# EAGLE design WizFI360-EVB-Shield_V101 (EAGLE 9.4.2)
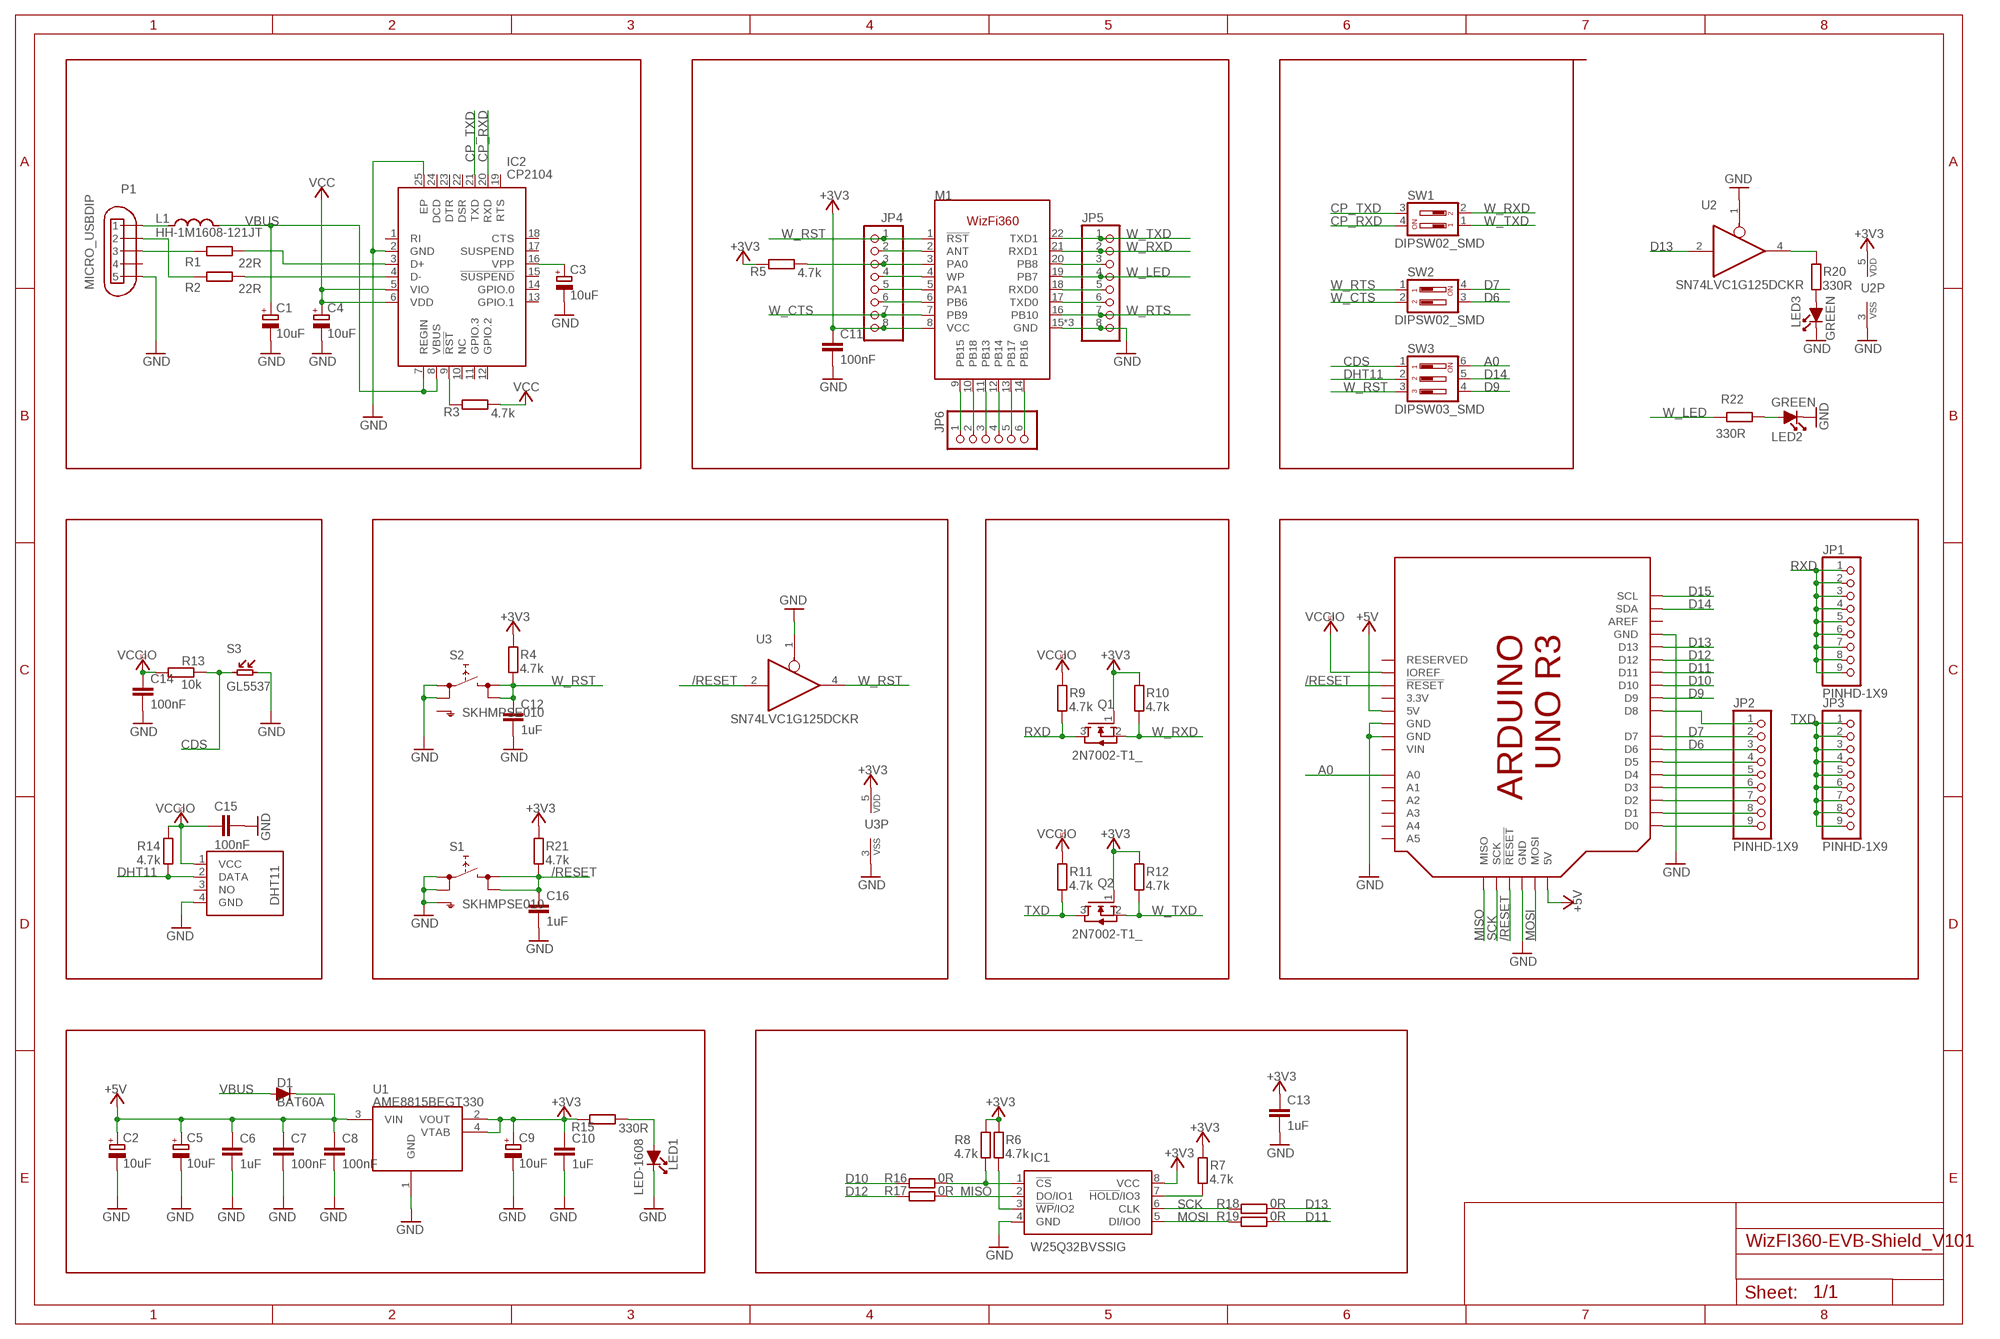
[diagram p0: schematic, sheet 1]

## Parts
C1  10uF  0474_TAJA475M016RNJ  [SMC_A]
C2  10uF  0474_TAJA475M016RNJ  [SMC_A]
C3  10uF  0474_TAJA475M016RNJ  [SMC_A]
C4  10uF  0474_TAJA475M016RNJ  [SMC_A]
C5  10uF  0474_TAJA475M016RNJ  [SMC_A]
C6  1uF  0142_10NF_0603  [C0603-ROUND@1]
C7  100nF  0142_10NF_0603  [C0603-ROUND@1]
C8  100nF  0142_10NF_0603  [C0603-ROUND@1]
C9  10uF  0474_TAJA475M016RNJ  [SMC_A]
C10  1uF  0142_10NF_0603  [C0603-ROUND@1]
C11  100nF  0142_10NF_0603  [C0603-ROUND@1]
C12  1uF  0142_10NF_0603  [C0603-ROUND@1]
C13  1uF  0142_10NF_0603  [C0603-ROUND@1]
C14  100nF  0142_10NF_0603  [C0603-ROUND@1]
C15  100nF  0142_10NF_0603  [C0603-ROUND@1]
C16  1uF  0142_10NF_0603  [C0603-ROUND@1]
D1  BAT60A  [BAT60A]
IC1  W25Q32BVSSIG  [SOIC127P790X216-8N]
IC2  CP2104  CP2104-F03-GMR  [QFN50P400X400X80-25N]
JP1  PINHD-1X9  [1X09]
JP2  PINHD-1X9  [1X09]
JP3  PINHD-1X9  [1X09]
JP4  PINHD-1X8  [1X08]
JP5  PINHD-1X8  [1X08]
JP6  PINHD-1X6  [1X06]
L1  HH-1M1608-121JT  BLM18PG471SN1D  [0603-1608X90N]
LED1  LED-1608  [LED-1608]
LED2  GREEN  LED-1608  [LED-1608]
LED3  GREEN  LED-1608  [LED-1608]
M1  WIZFI360  [WIZFI360]
M2  ARDUINO_R3_ICSP_5  [ARDUINOR3_ICSP_5]
P1  MICRO_USBDIP  [MICRO_USB_D]
Q1  2N7002-T1_  [SOT23]
Q2  2N7002-T1_  [SOT23]
R1  22R  0028_CR0603JW103L  [R0603-ROUND]
R2  22R  0028_CR0603JW103L  [R0603-ROUND]
R3  4.7k  0028_CR0603JW103L  [R0603-ROUND]
R4  4.7k  0028_CR0603JW103L  [R0603-ROUND]
R5  4.7k  0028_CR0603JW103L  [R0603-ROUND]
R6  4.7k  0028_CR0603JW103L  [R0603-ROUND]
R7  4.7k  0028_CR0603JW103L  [R0603-ROUND]
R8  4.7k  0028_CR0603JW103L  [R0603-ROUND]
R9  4.7k  0028_CR0603JW103L  [R0603-ROUND]
R10  4.7k  0028_CR0603JW103L  [R0603-ROUND]
R11  4.7k  0028_CR0603JW103L  [R0603-ROUND]
R12  4.7k  0028_CR0603JW103L  [R0603-ROUND]
R13  10k  0028_CR0603JW103L  [R0603-ROUND]
R14  4.7k  0028_CR0603JW103L  [R0603-ROUND]
R15  330R  0028_CR0603JW103L  [R0603-ROUND]
R16  0R  0028_CR0603JW103L  [R0603-ROUND]
R17  0R  0028_CR0603JW103L  [R0603-ROUND]
R18  0R  0028_CR0603JW103L  [R0603-ROUND]
R19  0R  0028_CR0603JW103L  [R0603-ROUND]
R20  330R  0028_CR0603JW103L  [R0603-ROUND]
R21  4.7k  0028_CR0603JW103L  [R0603-ROUND]
R22  330R  0028_CR0603JW103L  [R0603-ROUND]
S1  SKHMPSE010  [SKHMPXE010]
S2  SKHMPSE010  [SKHMPXE010]
S3  GL5537  [GL55]
S4  DHT11  [DHT11]
SW1  DIPSW02_SMD  [DIPSW02_SMD]
SW2  DIPSW02_SMD  [DIPSW02_SMD]
SW3  DIPSW03_SMD  [DIPSW03_SMD]
U1  AME8815BEGT330  [SOT-223]
U2  SN74LVC1G125DCKR  0040_SN74LVC1G125DCKR  [SC70-5]
U3  SN74LVC1G125DCKR  0040_SN74LVC1G125DCKR  [SC70-5]

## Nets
+3V3 [power]: C9.+ C10.1 C11.1 C13.1 IC1.8(VCC) JP4.8 M1.8(VCC) Q1.1(G) Q2.1(G) R4.1 R5.2 R6.1 R7.1 R8.1 R10.1 R12.1 R15.2 R21.1 U1.2(VOUT) U1.4(VTAB) U2.5(VDD) U3.5(VDD)
+5V [power]: C2.+ C5.+ C6.1 C7.1 C8.1 D1.1 M2.5V M2.5V_ICSP(5V) U1.3(VIN)
/RESET: C16.1 M2.RESET(!RESET!) M2.RESET_ICSP(!RESET) R21.2 S1.3(2.1) S1.4(2.2) U3.2(I)
A0: M2.A0 SW3.6
CDS: R13.2 S3.P$1 SW3.1
CP_RXD: IC2.20(RXD) SW1.4
CP_TXD: IC2.21(TXD) SW1.3
D6: JP2.3 M2.D6 SW2.3
D7: JP2.2 M2.D7 SW2.4
D9: M2.D9 SW3.4
D10: M2.D10 R16.1
D11: M2.D11 R19.2
D12: M2.D12 R17.1
D13: M2.D13 R18.2 U2.2(I)
D14: M2.SDA SW3.5
D15: M2.SCL
DHT11: R14.2 S4.2(DATA) SW3.2
GND: C1.- C2.- C3.- C4.- C5.- C6.2 C7.2 C8.2 C9.- C10.2 C11.2 C12.2 C13.2 C14.2 C15.2 C16.2 IC1.4(GND) IC2.2(GND) IC2.25(EP) JP5.8 LED1.K LED2.K LED3.K M1.15(GND) M1.23(GND) M1.24(GND) M2.GND M2.GND@1(GND) M2.GND@2(GND) M2.GND@3(GND) P1.5 P1.GND1 P1.GND2 P1.GND3 P1.GND4 P1.GND5 P1.GND6 S1.1(1.1) S1.2(1.2) S1.5(SH) S2.1(1.1) S2.2(1.2) S3.P$2 S4.4(GND) U1.1(GND) U2.1(OE) U2.3(VSS) U3.1(OE) U3.3(VSS)
MISO: IC1.2(DO/IO1) M2.MISO R17.2
MOSI: IC1.5(DI/IO0) M2.MOSI R19.1
N$1: L1.1 P1.1
N$2: IC2.4(D-) R2.1
N$3: IC2.3(D+) R1.1
N$4: P1.3 R1.2
N$5: P1.2 R2.2
N$6: C3.+ IC2.16(VPP)
N$7: LED1.A R15.1
N$8: IC2.9(!RST) R3.2
N$9: JP4.3 M1.3(PA0) R5.1
N$10: IC1.3(!WP!/IO2) R6.2
N$11: IC1.7(!HOLD!/IO3) R7.2
N$12: IC1.1(!CS) R8.2 R16.2
N$13: LED3.A R20.2
N$14: R20.1 U2.4(O)
N$15: JP2.1 M2.D8
N$17: LED2.A R22.2
N$18: JP2.4 M2.D5
N$19: JP2.5 M2.D4
N$20: JP2.6 M2.D3
N$21: JP2.7 M2.D2
N$22: JP2.8 M2.D1
N$23: JP2.9 M2.D0
N$24: JP4.2 M1.2(ANT)
N$25: JP4.4 M1.4(WP)
N$26: JP4.5 M1.5(PA1)
N$27: JP4.6 M1.6(PB6)
N$28: JP5.3 M1.20(PB8)
N$30: JP5.5 M1.18(RXD0)
N$31: JP5.6 M1.17(TXD0)
N$32: JP6.1 M1.9(PB15)
N$33: JP6.2 M1.10(PB18)
N$34: JP6.3 M1.11(PB13)
N$35: JP6.5 M1.13(PB17)
N$36: JP6.6 M1.14(PB16)
N$37: JP6.4 M1.12(PB14)
RXD: JP1.1 JP1.2 JP1.3 JP1.4 JP1.5 JP1.6 JP1.7 JP1.8 JP1.9 Q1.3(D) R9.2
SCK: IC1.6(CLK) M2.SCK R18.1
TXD: JP3.1 JP3.2 JP3.3 JP3.4 JP3.5 JP3.6 JP3.7 JP3.8 JP3.9 Q2.3(D) R11.2
VBUS: C1.+ D1.2 IC2.7(REGIN) IC2.8(VBUS) L1.2
VCC: C4.+ IC2.5(VIO) IC2.6(VDD) R3.1
VCCIO: C14.1 C15.1 M2.IOREF R9.1 R11.1 R13.1 R14.1 S4.1(VCC)
W_CTS: JP4.7 M1.7(PB9) SW2.2
W_LED: JP5.4 M1.19(PB7) R22.1
W_RST: C12.1 JP4.1 M1.1(!RST!) R4.2 S2.3(2.1) S2.4(2.2) SW3.3 U3.4(O)
W_RTS: JP5.7 M1.16(PB10) SW2.1
W_RXD: JP5.2 M1.21(RXD1) Q1.2(S) R10.2 SW1.2
W_TXD: JP5.1 M1.22(TXD1) Q2.2(S) R12.2 SW1.1
Unconnected: IC2.1(RI) IC2.10(NC) IC2.11(GPIO.3) IC2.12(GPIO.2) IC2.13(GPIO.1) IC2.14(GPIO.0) IC2.15(!SUSPEND) IC2.17(SUSPEND) IC2.18(CTS) IC2.19(RTS) IC2.22(DSR) IC2.23(DTR) IC2.24(DCD) M2.A1 M2.A2 M2.A3 M2.A4 M2.A5 M2.AREF M2.RESERVED P1.4 S2.5(SH) S4.3(NO)

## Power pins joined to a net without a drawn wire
3.3V: M2.3V(3.3V)
VIN: M2.VIN

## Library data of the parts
C1-C5 C9 = Condensatori:0474_TAJA475M016RNJ: 4u7 tantalio Case A - testa gialla -Tantalio; CASE: CaseA_(1206); MONTHLY_USAGE: _____; PART_NUMBER: TAJA475M016RNJ; PRICE: _____; SUPPLIER: _____; TYPE: Condensatori; VALUE: 4u7
C6-C8 C10-C16 = Condensatori:0142_10NF_0603: 10nF 0603; CASE: 0603; MONTHLY_USAGE: _____; PART_NUMBER: 10nF_0603; PRICE: _____; SUPPLIER: _____; TYPE: Condensatori; VALUE: 10nF
D1 = DIODE:BAT60A
IC1 = untitled:W25Q32BVSSIG: 3v 32Mbit Serial Flash with Dual and Quad SPI Source: Datasheet; DESCRIPTION: 3v 32Mbit Serial Flash with Dual and Quad SPI; HEIGHT: 2.16mm; MANUFACTURER_NAME: Winbond; MANUFACTURER_PART_NUMBER: W25Q32BVSSIG
IC2 = untitled:CP2104-F03-GMR: USB-to-UART 1-CH 576byte FIFO 3.3V Automotive 24-Pin QFN EP T/R Source: Datasheet; DESCRIPTION: USB-to-UART 1-CH 576byte FIFO 3.3V Automotive 24-Pin QFN EP T/R; HEIGHT: 0.8mm; MANUFACTURER_NAME: Silicon Labs; MANUFACTURER_PART_NUMBER: CP2104-F03-GMR; MOUSER_PART_NUMBER: 634-CP2104-F03-GMR; MOUSER_PRICE-STOCK: https://www.mouser.com/Search/Refine.aspx?Keyword=634-CP2104-F03-GMR
JP1-JP3 = PinHeader:PINHD-1X9
JP4 JP5 = PinHeader:PINHD-1X8: PIN HEADER
JP6 = PinHeader:PINHD-1X6: PIN HEADER
L1 = MK1_Zero:BLM18PG471SN1D: FERRITE CHIP 470 OHM 1000MA 0603
LED1-LED3 = DIODE:LED-1608
M1 = WIZnet:WIZFI360
M2 = Arduino:ARDUINO_R3_ICSP_5
P1 = Connector:MICRO_USB
Q1 Q2 = TRANSISTOR:2N7002-T1
R1-R12 R14-R22 = Resistenze:0028_CR0603JW103L: 10K 0603; CASE: 0603; MONTHLY_USAGE: _____; PART_NUMBER: CR0603JW103L; PRICE: _____; SUPPLIER: _____; TYPE: Resistenze; VALUE: 10k
R13 = Resistenze:0028_CR0603JW103L: 10K 0603; CASE: 0603; MONTHLY_USAGE: _____; PART_NUMBER: CR0603JW103L; PRICE: _____; SUPPLIER: _____; TYPE: Resistenze
S1 S2 = Switch:SKHMP*E010: 6.2 X 6.5mm TACT Switch (SMD) Source: http://www3.alps.co.jp/WebObjects/catalog.woa/PDF/E/Switch/Tact/SKHM/SKHM.PDF
S3 = misc:GL5537: GL5537 Photoresistor
S4 = DHT11:DHT11: DHT11 Czujnik temperatury i wilgotności
SW1 SW2 = Switch:DIPSW02_SMD
SW3 = Switch:DIPSW03_SMD
U1 = RECULATOR:AME8815BEGT330
U2 U3 = Circuito Integrato:0040_SN74LVC1G125DCKR: Single bus buffer with 3-state output; CASE: SC70; MONTHLY_USAGE: _____; PART_NUMBER: SN74LVC1G125DCKR; PRICE: _____; SPICEPREFIX: U; SUPPLIER: _____; TYPE: Circuito_Integrato; VALUE: 74LVC1G125DCKR

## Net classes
0 default: width 0.203 mm, drill 0.008 mm, clearance 0.127 mm
1 power: width 0.305 mm, drill 0.3 mm, clearance 0.203 mm
2 gnd: width 0.305 mm, drill 0.3 mm, clearance 0.127 mm

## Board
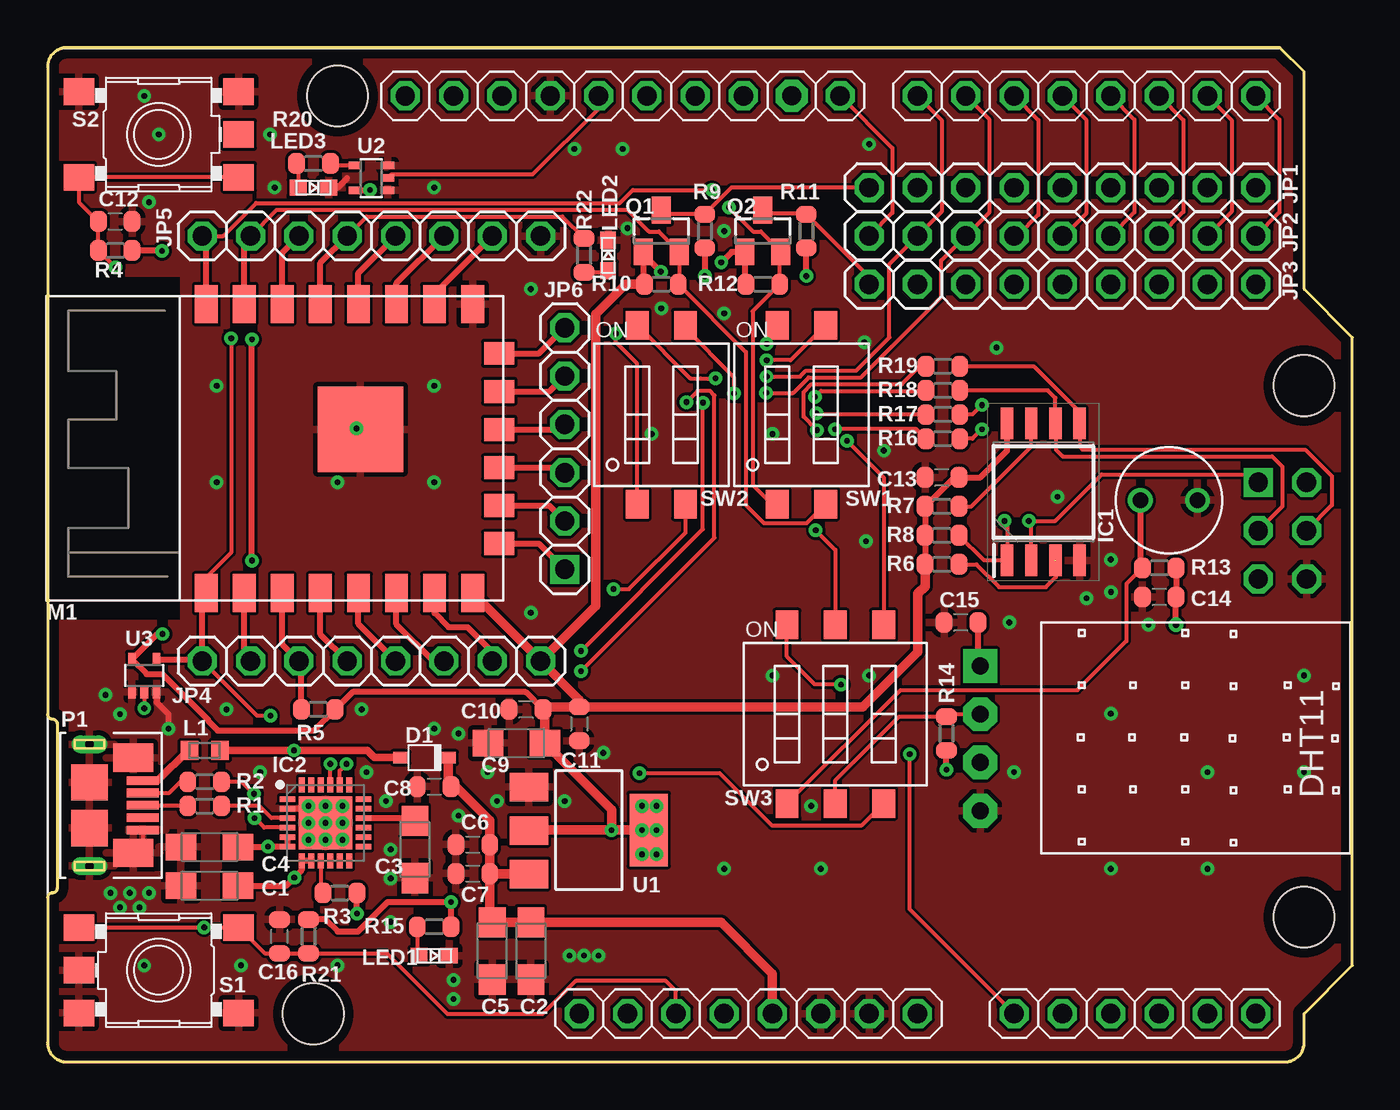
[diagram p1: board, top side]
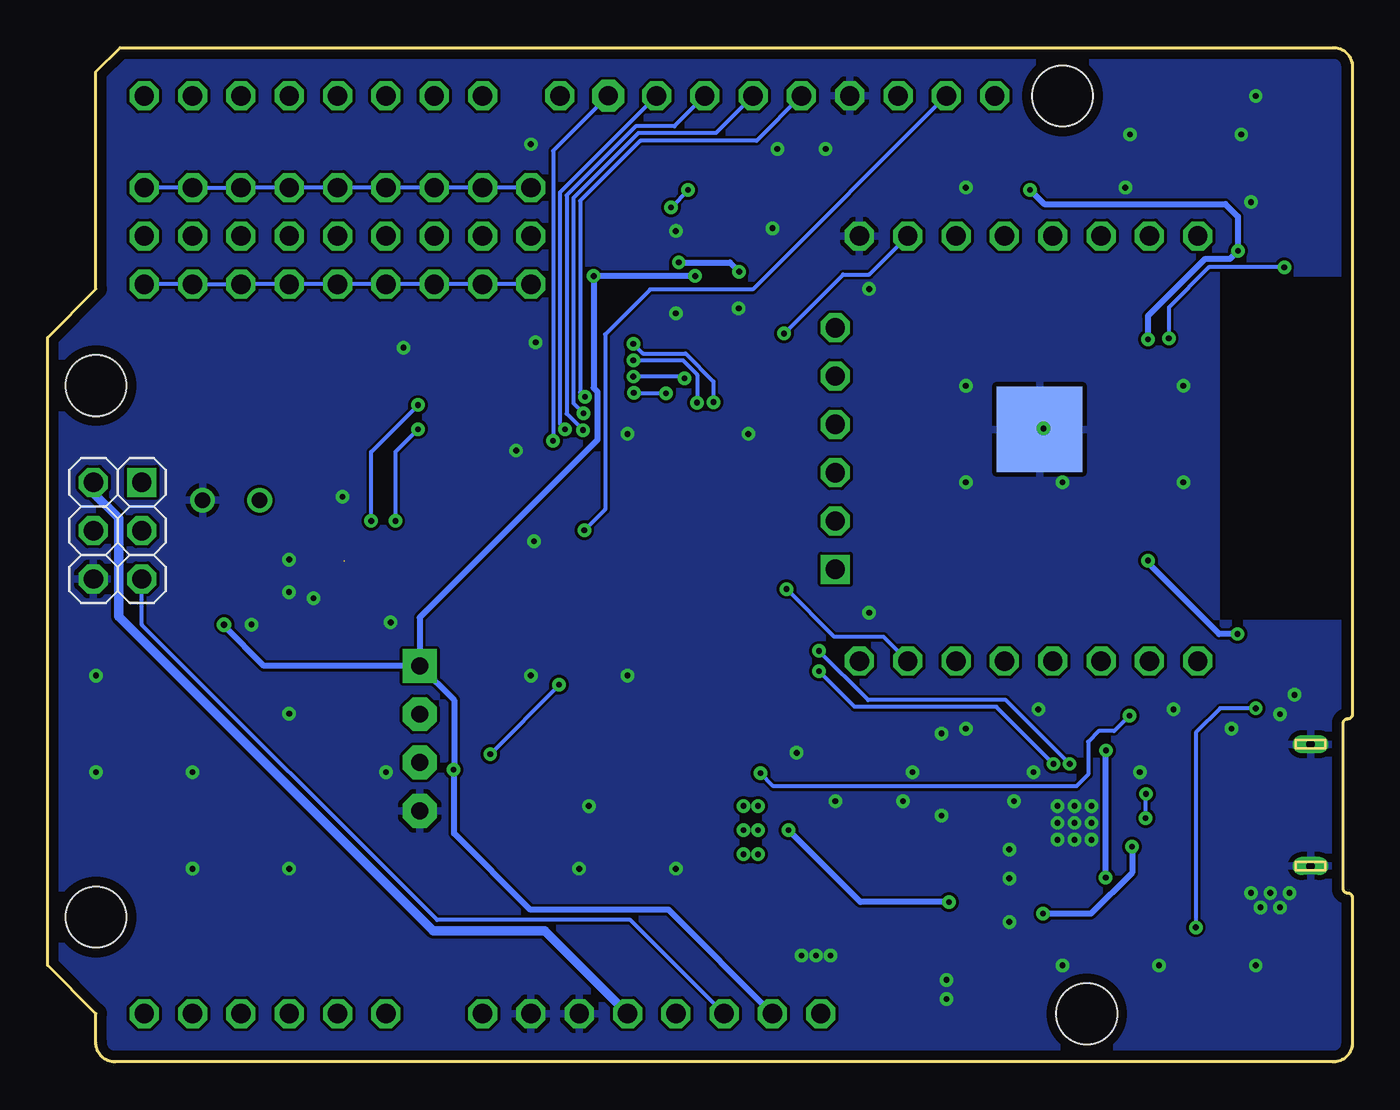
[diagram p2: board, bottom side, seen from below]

Size 68.58 x 53.34 mm. Coordinates in mm from the lower left corner, seen from the top.
Outline: 0.51,9.14 arc-90 0.25,8.89 arc90 0,8.64 0,1.02 arc90 1.02,0 65.02,0 arc90 66.04,1.02 66.04,2.54 68.58,5.08 68.58,38.1 66.04,40.64 66.04,52.07 64.77,53.34 1.02,53.34 arc90 0,52.32 0,18.29 arc90 0.25,18.03 arc-90 0.51,17.78 0.51,9.14
Copper layers (1*16): Top 0.035mm / dielectric 1.5mm / Bottom 0.035mm
Design rules "default *": minimum track width 6mil, minimum drill 0.3mm, track to track 6mil, track to pad 6mil, pad to pad 6mil, via to via 6mil, smd to smd 3mil, copper to edge 20mil, drill to drill 10mil, minimum pad ring 10mil, minimum via ring 8mil, stop-mask expansion 4mil, vias tented up to drill 15mil, thermal gap 10mil

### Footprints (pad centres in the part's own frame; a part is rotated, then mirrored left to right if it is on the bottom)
SMC_A = smd 1.6 x 1.4: + -1.5,0; - 1.5,0
C0603-ROUND@1 = smd 0.898 x 1.1: 1 -0.889,0; 2 0.889,0
BAT60A = smd 0.8 x 0.6: 1 1.25,0; 2 -1.25,0
SOIC127P790X216-8N = smd 1.65 x 0.65: 1 -3.6,1.905; 2 -3.6,0.635; 3 -3.6,-0.635; 4 -3.6,-1.905; 5 3.6,-1.905; 6 3.6,-0.635; 7 3.6,0.635; 8 3.6,1.905
QFN50P400X400X80-25N = smd 0.8 x 0.3: 1 -2,1.25; 2 -2,0.75; 3 -2,0.25; 4 -2,-0.25; 5 -2,-0.75; 6 -2,-1.25; 13 2,-1.25; 14 2,-0.75; 15 2,-0.25; 16 2,0.25; 17 2,0.75; 18 2,1.25 | smd 0.3 x 0.8: 7 -1.25,-2; 8 -0.75,-2; 9 -0.25,-2; 10 0.25,-2; 11 0.75,-2; 12 1.25,-2; 19 1.25,2; 20 0.75,2; 21 0.25,2; 22 -0.25,2; 23 -0.75,2; 24 -1.25,2 | smd 2.8 x 2.8: 25 0,0
1X09 = drill 1.016 octagon: 1 -11.43,0; 2 -8.89,0; 3 -6.35,0; 4 -3.81,0; 5 -1.27,0; 6 1.27,0; 7 3.81,0; 8 6.35,0; 9 8.89,0
1X08 = drill 1.016 octagon: 1 -8.89,0; 2 -6.35,0; 3 -3.81,0; 4 -1.27,0; 5 1.27,0; 6 3.81,0; 7 6.35,0; 8 8.89,0
1X06 = drill 1.016 square: 1 -6.35,0 | drill 1.016 octagon: 2 -3.81,0; 3 -1.27,0; 4 1.27,0; 5 3.81,0; 6 6.35,0
0603-1608X90N = smd 0.95 x 1: 1 -0.8,0; 2 0.8,0
LED-1608 = smd 0.89 x 0.82: A -0.8,0; K 0.8,0
WIZFI360 = smd 2 x 1.2: 1 -7.6,3.6; 2 -7.6,1.6; 3 -7.6,-0.4; 4 -7.6,-2.4; 5 -7.6,-4.4; 6 -7.6,-6.4; 7 -7.6,-8.4; 8 -7.6,-10.4; 15 7.6,-10.4; 16 7.6,-8.4; 17 7.6,-6.4; 18 7.6,-4.4; 19 7.6,-2.4; 20 7.6,-0.4; 21 7.6,1.6; 22 7.6,3.6 | smd 1.2 x 1.6: 9 -5,-11.8; 10 -3,-11.8; 11 -1,-11.8; 12 1,-11.8; 13 3,-11.8; 14 5,-11.8 | smd 4.5 x 4.5: 23 1,-4.5 | smd 4.5 x 4.5 bottom: 24 1,-4.5
ARDUINOR3_ICSP_5 = drill 1.016 octagon: 3V 35.56,2.54; 5V 38.1,2.54; 5V_ICSP 66.167,30.48; A0 50.8,2.54; A1 53.34,2.54; A2 55.88,2.54; A3 58.42,2.54; A4 60.96,2.54; A5 63.5,2.54; AREF 23.876,50.8; D0 63.5,50.8; D1 60.96,50.8; D2 58.42,50.8; D3 55.88,50.8; D4 53.34,50.8; D5 50.8,50.8; D6 48.26,50.8; D7 45.72,50.8; D8 41.656,50.8; D10 36.576,50.8; D11 34.036,50.8; D12 31.496,50.8; D13 28.956,50.8; GND 26.416,50.8; GND@1 43.18,2.54; GND@2 40.64,2.54; GND@3 66.167,25.4; IOREF 30.48,2.54; MOSI 66.167,27.94; RESERVED 27.94,2.54; RESET 33.02,2.54; RESET_ICSP 63.627,25.4; SCK 63.627,27.94; SCL 18.796,50.8; SDA 21.336,50.8; VIN 45.72,2.54 | drill 1 pad 1.676 octagon: D9 39.116,50.8 | drill 1.016 square: MISO 63.627,30.48 | hole 3.2: 66.04,7.62; 66.04,35.56; 15.24,50.8; 13.97,2.54
MICRO_USB_D = smd 1.7 x 0.45: 1 2.8,1.3; 2 2.8,0.65; 3 2.8,0; 4 2.8,-0.65; 5 2.8,-1.3 | drill 0.45 long: GND1 0,3.2; GND4 0,-3.2 | smd 2.1 x 1.475: GND2 2.3,2.5; GND3 2.3,-2.5 | smd 1.9 x 1.9: GND5 0,-1.2; GND6 0,1.2
SOT23 = smd 1 x 1.4: 1 -0.95,-1.1; 2 0.95,-1.1; 3 0,1.1
R0603-ROUND = smd 0.898 x 1.1: 1 -0.889,0; 2 0.889,0
SKHMPXE010 = smd 1.6 x 1.4: 1 -4.2,2.25; 2 4.2,2.25; 3 -4.2,-2.25; 4 4.2,-2.25; 5 4.2,0
GL55 = drill 0.8: P$1 -1.5,0; P$2 1.5,0
DHT11 = drill 0.889 pad 1.778 square: 1 -3.81,-11.43 | drill 0.889 pad 1.778 octagon: 2 -1.27,-11.43; 3 1.27,-11.43; 4 3.81,-11.43
DIPSW02_SMD = smd 1.2 x 1.5: 1 -1.27,-4.7; 2 1.27,-4.7; 3 1.27,4.7; 4 -1.27,4.7
DIPSW03_SMD = smd 1.2 x 1.5: 1 -2.54,-4.7; 2 0,-4.7; 3 2.54,-4.7; 4 2.54,4.7; 5 0,4.7; 6 -2.54,4.7
SOT-223 = smd 1.499 x 2.007: 1 -2.261,-3.15; 2 0.025,-3.15; 3 2.311,-3.15 | smd 3.81 x 2.007: 4 0,3.15
SC70-5 = smd 0.4 x 0.7: 1 -0.65,-0.85; 2 0,-0.85; 3 0.65,-0.85; 4 0.65,0.85; 5 -0.65,0.85

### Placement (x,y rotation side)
C1  8.51,9.27 180 top
C2  25.4,5.84 270 top
C3  19.3,11.18 270 top
C4  8.51,11.3 180 top
C5  23.37,5.84 270 top
C6  22.35,11.43 180 top
C7  22.35,9.91 180 top
C8  20.32,14.48 180 top
C9  24.64,16.76 180 top
C10  25.15,18.54 180 top
C11  27.94,17.78 270 top
C12  3.56,44.2 0 top
C13  47.01,30.74 180 top
C14  58.43,24.46 180 top
C15  48.01,23.11 180 top
C16  12.19,6.6 90 top
D1  19.81,16 0 top
IC1  52.33,29.97 90 top
IC2  14.61,12.57 0 top
JP1  54.61,45.97 0 top
JP2  54.61,43.43 0 top
JP3  54.61,40.89 0 top
JP4  17.02,21.08 0 top
JP5  17.02,43.43 0 top
JP6  27.18,32.26 90 top
L1  8.26,16.38 0 top
LED1  20.32,5.59 0 top
LED2  29.46,42.42 90 top
LED3  13.97,45.97 0 top
M1  11.94,32.26 90 top
M2  0,0 0 top
P1  2.2,13.5 0 top
Q1  32.26,43.69 0 top
Q2  37.59,43.69 0 top
R1  8.26,13.46 180 top
R2  8.26,14.73 180 top
R3  15.37,8.89 180 top
R4  3.56,42.67 180 top
R5  14.22,18.54 0 top
R6  47.01,26.17 0 top
R7  47.01,29.22 0 top
R8  47.01,27.69 0 top
R9  34.54,43.69 90 top
R10  32.26,40.89 0 top
R11  39.88,43.69 90 top
R12  37.59,40.89 0 top
R13  58.43,25.98 180 top
R14  47.24,17.27 90 top
R15  20.32,7.11 0 top
R16  47.05,32.77 0 top
R17  47.05,34.04 0 top
R18  47.05,35.31 180 top
R19  47.05,36.58 180 top
R20  13.97,47.24 180 top
R21  13.72,6.6 270 top
R22  28.19,42.42 270 top
S1  5.84,4.83 180 top
S2  5.84,48.77 0 top
S3  58.94,29.54 0 top
S4  60.45,17.02 270 top
SW1  39.62,34.04 0 top
SW2  32.26,34.04 0 top
SW3  41.4,18.29 0 top
U1  28.45,12.19 270 top
U2  17.02,46.48 90 top
U3  5.08,20.32 0 top
U$2  [WIZFI_LOGO]  47,15 0 bottom

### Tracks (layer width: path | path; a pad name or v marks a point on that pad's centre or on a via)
+3V3  (via drill 0.3)
  Top 0.305: R12.1 36.64,40.95 Q2.1 35.96,42.59 v35.41,42.04 | R10.1 31.31,40.95 Q1.1 31.31,42.48 v32.23,41.55 | IC1.8 50.43,32.14 49.03,30.74 C13.1 47.64,30.74 R7.1 R8.1 R6.1 | C10.1 25.12,19.46 16.03,19.46 R5.2 13.99,17.42 8.94,17.42 8.46,17.91 8.46,17.96 6.02,20.4 5.2,20.4 U3.5 5.76,22.5 v6.04,22.5 | v6.02,42.65 5.99,42.67 R4.1 | v10.74,26.36 v10.74,38 | U2.5 16.93,45.83 v16.94,45.85 | U1.4 31.6,11.33 v32,10.92 | v32,13.46 31.6,13.06 U1.4 | U1.4 v32,12.19 | U1.4 31.6,13.11 v31.24,13.46 | R21.1 14.61,7.49 15.24,6.86 16.32,6.86 17.87,8.41 v21.21,8.41 R15.2
  Top 0.406: v31.24,10.92 31.24,11.84 U1.4 v31.24,12.19
  Top 0.508: v31.24,12.19 v29.64,12.19 | v29.64,12.19 25.32,12.19 U1.2 | 29.69,12.24 v29.64,12.19 | 26.04,16.87 C9.+ | v29.64,12.19 29.64,13.26 C9.+ | C9.+ 26.14,18.44 C10.1 26.16,18.67 C11.1 | C11.1 27.94,19.05 JP4.8 | C11.1 42.85,18.67 45.74,21.57 45.74,24.64 46.12,25.01 R6.1 | JP4.8 28.8,23.98 28.8,39.32 30.38,40.89 R10.1 | M1.8 22.73,24.26 JP4.8
  Bottom 0.305: v35.41,42.04 32.72,42.04 v32.23,41.55 | v6.04,22.5 7.01,22.5 10.74,26.24 v10.74,26.36 | v10.74,38 10.74,39.22 10.75,39.22 7.73,42.24 6.43,42.24 v6.02,42.65 6.02,44.45 6.68,45.11 16.2,45.11 v16.94,45.85 | v29.64,12.19 25.86,8.41 v21.21,8.41 21.21,8.38
+5V
  Top 0.508: D1.1 21.06,14.62 C8.1 21.46,14.48 23.24,12.7 C6.1 C7.1 | C7.1 23.24,7.47 C5.+ C2.+ 35.41,7.34 38.1,4.65 M2.5V | C7.1 23.27,9.88 U1.3
  Bottom 0.508: M2.5V 42.44,6.88 48.31,6.88 64.85,23.42 64.85,28.6 66.17,29.92 M2.5V_ICSP
/RESET  (via drill 0.3)
  Top 0.203: S1.4 v8.23,7.08 S1.3 | M2.RESET 33.02,3.73 32.49,4.27 27.76,4.27 26.01,2.52 21.03,2.52 17.83,5.71 R21.2 C16.1 11.4,5.71 S1.3 | 10.16,6.96 S1.3 | U3.2 v5.08,18.59
  Bottom 0.203: v5.08,18.59 6.96,18.59 8.23,17.32 v8.23,7.08 | M2.RESET 37.95,7.47 48.11,7.47 63.63,22.99 M2.RESET_ICSP
A0  (via drill 0.3)
  Top 0.203: M2.A0 45.31,8.03 v45.31,16.18 | v41.71,19.84 41.68,19.86 40.31,19.86 38.86,21.31 SW3.6
  Bottom 0.203: v45.31,16.18 41.71,19.79 v41.71,19.84
CDS
  Top 0.203: SW3.1 44.83,19.56 54.13,19.56 56.7,22.13 56.7,25.14 R13.2
  Top 0.305: S3.P$1 57.44,26.08 R13.2
CP_RXD  (via drill 0.3)
  Top 0.203: SW1.4 37.8,38.18 v37.8,37.76 | IC2.20 15.36,15.31 v15.72,15.67 | v28.04,20.55 35.05,27.56 35.05,35.05 34.83,35.28 34.16,35.28 v33.58,34.7
  Bottom 0.203: v37.8,37.76 37.29,37.25 35.05,37.25 33.58,35.79 v33.58,34.7 | v15.72,15.67 18.71,18.67 26.16,18.67 v28.04,20.55
CP_TXD  (via drill 0.3)
  Top 0.203: SW1.3 39.05,36.9 v37.8,36.9 | IC2.21 v14.86,15.67 | v28.04,21.61 34.44,28.02 v34.44,34.67
  Bottom 0.203: v37.8,36.9 35.2,36.9 34.44,36.14 v34.44,34.67 | v14.86,15.67 18.21,19.02 25.45,19.02 v28.04,21.61
D6  (via drill 0.3)
  Top 0.203: M2.D6 49.48,49.58 49.48,44.65 JP2.3 46.97,42.14 46.97,40.21 42.75,35.99 40,35.99 39.18,35.18 v37.77,35.18 | SW2.3 33.53,38.56 36.07,36.01 v36.07,35.15
  Bottom 0.203: v37.77,35.18 36.1,35.18 v36.07,35.15
D7  (via drill 0.3)
  Top 0.203: M2.D7 46.99,49.53 46.99,44.7 JP2.2 44.25,41.96 44.25,38.1 42.49,36.35 39.85,36.35 39.54,36.04 v37.8,36.04 | SW2.4 33.78,35.95 34.31,35.95 v35.1,35.95
  Bottom 0.203: v35.1,35.95 35.2,36.04 v37.8,36.04
D9  (via drill 0.3)
  Top 0.203: v42.01,32.67 43.94,30.74 SW3.4
  Bottom 0.203: M2.D9 42.01,47.9 v42.01,32.67
D10  (via drill 0.3)
  Top 0.203: R16.1 45.66,33.27 v41.38,33.27
  Bottom 0.203: M2.D10 41.66,45.72 41.66,33.55 v41.38,33.28 v41.38,33.27
D11  (via drill 0.3)
  Top 0.203: v40.44,33.22 39.73,33.93 39.73,35.22 40.14,35.64 44.9,35.64 45.84,36.58 R19.2
  Bottom 0.203: M2.D11 35.64,49.2 37.67,49.2 41.3,45.57 41.3,34.09 v40.44,33.22
D12  (via drill 0.3)
  Top 0.203: R17.1 40.48,34.04 v40.41,34.11
  Bottom 0.203: M2.D12 33.45,48.84 37.53,48.84 40.95,45.42 40.95,34.65 v40.41,34.11
D13  (via drill 0.3)
  Top 0.203: v40.34,34.97 40.65,35.28 46.13,35.28 R18.2 | U2.2 18.06,46.68 25.5,46.68 28.96,50.13 M2.D13
  Bottom 0.203: M2.D13 31.32,48.44 37.43,48.44 40.59,45.28 40.59,35.22 v40.34,34.97
D14  (via drill 0.3)
  Top 0.203: v40.37,27.95 41.4,26.92 SW3.5
  Bottom 0.203: M2.SDA 31.52,40.62 36.91,40.62 39.27,38.25 39.27,29.05 v40.37,27.95
DHT11
  Top 0.203: S4.2 47.37,18.29 R14.2 44.76,18.16 41.4,14.81 SW3.2
GND  (via drill 0.3)
  Top 0.203: P1.5 5,11.5 P1.GND3
  Top 0.305: LED3.K 15.24,45.97 15.75,46.48 | IC2.2 13.58,13.32 v13.72,13.46 | U3.3 5.73,18.91 6.35,18.29 v6.35,17.53
  other vias: 15.49,13.46 13.72,11.68 15.49,11.68 14.61,13.46 13.72,12.57 15.49,12.57 14.61,11.68 14.61,12.57 5.08,5.08 10.16,5.08 15.24,5.08 60.96,10.16 55.88,10.16 40.64,10.16 35.56,10.16 50.8,15.24 60.96,15.24 66.04,15.24 66.04,20.32 55.88,18.32 38.1,20.32 15.24,30.48 16.24,33.31 20.32,35.56 20.32,30.48 25.4,40.64 5.08,50.8 20.32,45.97 49.88,37.56 43.02,27.38 57.86,23 21.59,17.27 23.62,13.72 17.78,13.72 18.03,9.65 21.34,4.32 27.43,5.59 28.19,5.59 28.96,5.59 27.18,13.72 29.21,16.26 11.18,15.24 5.33,8.89 4.32,8.89 3.3,8.89 4.83,8.13 3.81,8.13 21.34,3.3 9.4,18.54 8.89,30.48 8.89,35.56 11.68,48.77 5.84,48.77 5.33,45.21 55.88,26.42 55.9,24.71 54.61,24.38 50.55,23.11 27.69,48.01 30.23,48.01 43.18,48.26 43.95,32.15 35.56,39.37 31.75,33.02 38.1,33.02 43.18,20.32 18.03,7.37 3.81,18.29 3.05,19.3 25.4,23.62 32.26,39.62 53.09,29.72 42.93,37.85 35.56,43.69 30.48,43.84 40.13,13.46 20.32,17.53 16.51,18.54 16.76,15.24 18.03,11.18 21.59,12.95 23.11,15.24 11.94,45.97
  pour Top: -1.27,-1.27 69.85,-1.27 69.85,54.61 -1.27,54.61
  pour Bottom: -2.54,-2.54 -2.54,55.88 71.12,55.88 71.12,-2.54
MISO  (via drill 0.3)
  Top 0.203: IC1.2 51.7,28.32 v51.57,28.45 52.95,28.45 55.4,30.9 63.21,30.9 M2.MISO | v49.11,34.54 48.61,34.04 R17.2
  Bottom 0.203: v51.57,28.45 51.57,32.08 v49.11,34.54
MOSI
  Top 0.203: R19.1 51.82,36.58 54.24,34.17 IC1.5 54.24,32.36 54.4,32.2 66.1,32.2 67.5,30.8 67.5,29.27 M2.MOSI
N$1
  Top 0.406: P1.1 5.8,14.8 7.38,16.38 L1.1
N$2  (via drill 0.3)
  Top 0.203: IC2.4 11.38,12.32 v10.87,12.82 | v10.85,14.1 10.21,14.73 R2.1
  Bottom 0.203: v10.87,12.82 10.87,14.07 v10.85,14.1
N$3
  Top 0.203: IC2.3 11.76,12.82 11.12,13.46 R1.1
N$4
  Top 0.203: 7.33,13.5 R1.2 5.04,13.46 P1.3
N$5
  Top 0.203: P1.2 6.4,14.15 6.98,14.73 R2.2
N$6
  Top 0.305: IC2.16 19.16,12.82 C3.+
N$7
  Top 0.203: R15.1 19.43,5.68 LED1.A
N$8
  Top 0.203: IC2.9 14.36,9.01
  Top 0.305: 14.36,9.01 R3.2
N$9
  Top 0.305: R5.1 13.34,20.95 JP4.3 12.34,21.95 M1.3
N$10  (1 unrouted)
  Top 0.203: R6.2 48.81,26.17 50.01,24.97 52.47,24.97 53,25.5 53,26.34
N$11
  Top 0.203: R7.2 48.55,29.22 51.7,32.36 IC1.7
N$12  (via drill 0.3)
  Top 0.203: R8.2 49.22,26.37 IC1.1 50.43,28.32 v50.3,28.45 | v49.11,33.27 48.61,32.77 R16.2
  Bottom 0.203: v49.11,33.27 50.3,32.08 v50.3,28.45
N$13
  Top 0.203: R20.2 13.17,47.16 LED3.A
N$14
  Top 0.203: U2.4 14.97,47.13 R20.1
N$15
  Top 0.203: M2.D8 44.4,48.06 44.4,44.65 JP2.1
N$17
  Top 0.203: R22.2 29.38,41.53 LED2.A
N$18
  Top 0.203: M2.D5 52.07,49.53 52.07,44.55 50.95,43.43 JP2.4
N$19
  Top 0.203: M2.D4 54.59,49.55 54.59,44.6 53.42,43.43 JP2.5
N$20
  Top 0.203: M2.D3 57.12,49.55 57.12,44.68 JP2.6
N$21
  Top 0.203: M2.D2 59.69,49.53 59.69,44.7 JP2.7
N$22
  Top 0.203: M2.D1 62.23,49.53 62.23,44.7 JP2.8
N$23
  Top 0.203: M2.D0 64.75,49.55 64.75,44.68 JP2.9
N$24
  Top 0.305: JP4.2 10.34,21.41 M1.2
N$25
  Top 0.305: JP4.4 14.34,22.49 M1.4
N$26
  Top 0.305: JP4.5 16.34,23.03 M1.5
N$27
  Top 0.305: JP4.6 20.27,21.08 18.34,23.01 M1.6
N$28
  Top 0.305: M1.20 12.34,42.56 JP5.3
N$30
  Top 0.305: M1.18 16.34,41.48 JP5.5
N$31
  Top 0.305: M1.17 18.34,40.94 JP5.6
N$32
  Top 0.305: M1.9 25.83,27.26 JP6.1
N$33
  Top 0.305: M1.10 26.37,29.26 JP6.2
N$34
  Top 0.305: M1.11 26.91,31.26 JP6.3
N$35
  Top 0.305: M1.13 26.37,35.26 JP6.5
N$36
  Top 0.305: M1.14 25.83,37.26 JP6.6
N$37
  Top 0.305: M1.12 26.91,33.26 JP6.4
RXD
  Top 0.203: JP1.1 35.94,45.97 R9.2 32.47,44.58 Q1.3
  Bottom 0.203: JP1.1 JP1.2 JP1.3 JP1.4 JP1.5 JP1.6 JP1.7 JP1.8 JP1.9
SCK
  Top 0.203: R18.1 52.57,35.31 52.97,34.92 IC1.6 53,33.54 53,32.2 53.36,31.84 64.36,31.84 64.9,31.3 64.9,29.21 M2.SCK
TXD
  Top 0.203: Q2.3 37.77,44.61 39.84,44.61 R11.2 43.18,41.27 JP3.1
  Bottom 0.203: JP3.1 JP3.2 JP3.3 JP3.4 JP3.5 JP3.6 JP3.7 JP3.8 JP3.9
VBUS  (via drill 0.3)
  Top 0.305: C1.+ 12.55,9.27 v12.97,9.69 13.36,10.08 IC2.7 IC2.8
  Top 0.406: L1.2 v12.95,16.38 16.79,16.38 17.17,16 D1.2
  Bottom 0.305: v12.97,9.69 12.95,9.7 v12.95,16.38
VCC  (via drill 0.3)
  Top 0.305: C4.+ 10.03,11.32 v11.58,11.32 IC2.6 IC2.5 | v16.26,7.8 R3.1
  Bottom 0.305: v11.58,11.32 11.58,9.96 13.74,7.8 v16.26,7.8
VCCIO  (via drill 0.3, 0.35)
  Top 0.305: C15.1 48.9,20.95 S4.1 | 59.32,24.6 R13.1 59.34,25.95 | 59.32,24.6 C14.1 | R9.1 v34.54,41.33 | v39.88,41.33 R11.1 | v47.24,15.37 R14.1 | v59.3,23 59.3,24.58 59.32,24.6
  Bottom 0.305: v34.54,41.33 v39.88,41.33 39.88,35.44 39.68,35.24 39.68,32.71 49.02,23.37 S4.1 | M2.IOREF 35.94,8 43.2,8 47.22,12.01 47.22,15.37 | S4.1 47.22,19.02 47.22,15.37 | 47.22,15.37 v47.24,15.37 | S4.1 57.21,20.83 59.3,22.91 v59.3,23
W_CTS  (via drill 0.3)
  Top 0.203: v29.74,24.87 30.56,24.87 33.53,27.84 SW2.2
  Top 0.305: JP4.7 23.37,21.57 22.07,22.86 21.08,22.86 20.34,23.6 M1.7
  Bottom 0.203: JP4.7 24.64,22.35 27.23,22.35 v29.74,24.87
W_LED
  Top 0.203: JP5.4 16.76,44.45 27.05,44.45 R22.1
  Top 0.305: M1.19 14.34,42.02 JP5.4
W_RST  (via drill 0.3)
  Top 0.203: S2.4 S2.3 1.64,45.22 C12.1 R4.2 3.56,41.78 v3.58,41.78 | v9.65,38.05 9.65,26.8 8.34,25.48 M1.1 | JP4.1 11,18.21 v11.71,18.21 | v31.11,15.19 35.31,15.19 38.05,12.45 42.8,12.45 SW3.3
  Top 0.305: U3.4 8.04,21.17 JP4.1 8.13,24.05 M1.1
  Bottom 0.203: v3.58,41.78 7.54,41.78 9.65,39.67 v9.65,38.05 | v11.71,18.21 12.52,17.4 13.34,17.4 13.89,16.84 13.89,15.11 14.5,14.5 30.43,14.5 v31.11,15.19
W_RTS  (via drill 0.3)
  Top 0.203: SW2.1 30.99,36.73 29.87,37.85 v29.87,38.3
  Top 0.305: M1.16 20.34,40.4 JP5.7
  Bottom 0.203: v29.87,38.3 26.77,41.4 25.4,41.4 JP5.7
W_RXD
  Top 0.203: SW1.2 39.89,28.33 37.65,28.33 36.7,29.28 36.7,37.34 R10.2 33.21,40.95 Q1.2 32.13,43.66 31.6,43.66 30.45,44.81 12.04,44.81 JP5.2 10.92,43.69
  Top 0.305: M1.21 10.34,43.1 10.92,43.69
W_TXD  (via drill 0.3)
  Top 0.203: SW1.1 38.05,29.34 37.06,30.33 37.06,39.47 R12.2 38.48,42.53 Q2.2 38.54,42.61 37.49,43.66 37.08,43.66 v35.81,44.93 | JP5.1 9.23,43.43 10.96,45.16 30.07,45.16 30.76,45.85 v34.92,45.85
  Top 0.305: M1.22 8.34,43.22 JP5.1
  Bottom 0.203: v34.92,45.85 34.91,45.83 v35.81,44.93

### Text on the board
silk_top: WiFi RESET | JP10 | JP9 | SCL | SDA | AREF | GND | D13 | D12 | D11 | D10 | D9 | D8 | D7 | D6 | D5 | D4 | D3 | D2 | D1 | D0 | RXD | TXD | D8 | D7 | D6 | D5 | D4 | D3 | D2 | D1 | D0 | S3 | JP11 | <SW2> / RTS,CTS Sel / ON : D6, D7 / OFF : NC | <SW1> / RXD,TXD Sel / ON : USB / OFF:Arduino | S4 | <SW3> Pin Sel / 1:A0-CDS / 2:D14-DHT11 / 3:D9-WiFi RST / ON:Connect / OFF:NC | WizFI360-EVB-Shield | IOREF | RESET | 3.3V | 5V | GND | GND | VIN | A0 | A1 | A2 | A3 | A4 | A5 | RESET | JP7 | JP8
silk_bottom: SCL | SDA | AREF | GND | D13 | D12 | D11 | D10 | D9 | D8 | D7 | D6 | D5 | D4 | D3 | D2 | D1 | D0 | UART Sel Jumper | JP1 : RXD / JP2 : Arduino PIN / JP3 : TXD | Can't use to D6/D7, / If SW6 ON. | DIP Switch Information | <SW1> - UART RXD/TXD Selector / ON : Connect to USB / OFF : Connect to Arduino PIN(JP1 ,JP3) | <SW2> - UART RTS/CTS Selector / ON : Connect to Arduino PIN(D6 , D7) / OFF : Not Connect (Default) | <SW3> - Digital/Analog PIN Selector / 1 : A0 - CDS / 2 : D14 - DHT11 / 3 : D9 - WiFi Reset / ON : Connect to Arduino PIN / OFF : Not Connect (Default) | Board Model | WizFI360-EVB-Shield | Board Version | V1.01 | http://www.wiznet.io | Designed by WIZnet | Made in KOREA | IOREF | RESET | 3.3V | 5V | GND | GND | VIN | A0 | A1 | A2 | A3 | A4 | A5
